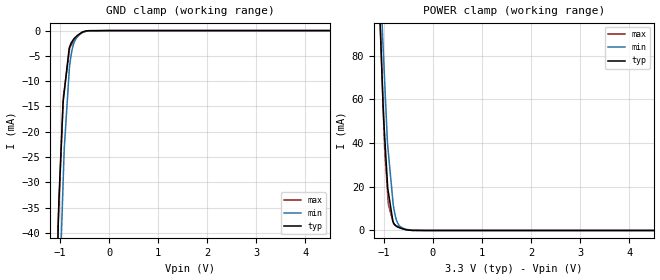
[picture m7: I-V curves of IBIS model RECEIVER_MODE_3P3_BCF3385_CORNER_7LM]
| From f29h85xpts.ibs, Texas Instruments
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|   Model Cell RECEIVER_MODE_3P3_BCF3385_CORNER_7LM
|RECEIVER_MODE_3P3_BCF3385_CORNER_7LM
[Model]   RECEIVER_MODE_3P3_BCF3385_CORNER_7LM
Model_type   Input
Polarity   Non-Inverting
Vinl = 0.8
Vinh = 2
|   typ   min   max
C_comp   0.44pF   0.4pF   0.46pF
[Model Spec]
Vinl   0.8   0.8   0.8
Vinh   2   2   2
[Temperature Range]   25   155   -40
[Voltage Range]   3.3   2.8   3.63
| Nom Voltages:
|   BIASFET=3.3, VDD=1.23, VDDS=3.3, VSS=0
| Min Voltages:
|   BIASFET=2.97, VDD=1.08, VDDS=2.8, VSS=0
| Max Voltages:
|   BIASFET=3.63, VDD=1.32, VDDS=3.63, VSS=0
[Power Clamp Reference]   3.3   2.8   3.63
[GND Clamp Reference]   0   0   0
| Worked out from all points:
|   GND clamp passes 1 mA (typ) near -0.65 V on its own axis
|   POWER clamp passes 1 mA (typ) near -0.65 V on its own axis
[GND Clamp]
|   Voltage   I(typ)   I(min)   I(max)
-3.3V     -1.475A    -1.211A    -2.162A
-1.048V   -42.88mA   -65.54mA   -41.3mA
-1.04V    -39.44mA   -62.35mA   -38.3mA
-1.024V   -33.44mA   -55.88mA   -34.51mA
-1.014V   -31.22mA   -52.39mA   -32.21mA
-939.5mV  -14.22mA   -30.38mA   -14.59mA
-932.9mV  -13.65mA   -28.43mA   -13.02mA
-915.9mV  -12.18mA   -23.39mA   -11.76mA
-809.2mV  -3.335mA   -7.228mA   -3.882mA
-719mV    -1.639mA   -2.468mA   -2.064mA
-549.8mV  -308.1uA   -409.6uA   -416.2uA
6.6V      0A         0A         0A
[POWER Clamp]
|   Voltage   I(typ)   I(min)   I(max)
-3.3V     1.946A     2.25A      2.109A
-1.078V   96.46mA    126.5mA    98.3mA
-1.036V   70.36mA    96.01mA    71.2mA
-1.025V   63.19mA    88.83mA    63.76mA
-1.004V   51.08mA    78.41mA    50.11mA
-979.4mV  41.74mA    66.36mA    35.51mA
-926.1mV  21.32mA    40.02mA    18.03mA
-906.9mV  17.35mA    35.39mA    11.76mA
-809.2mV  3.862mA    11.76mA    3.593mA
-746.4mV  1.971mA    5.025mA    2.171mA
-662.2mV  1.073mA    1.716mA    1.272mA
6.6V      0A         0A         0A
